FUNCTION "Uscite" : VOID
TITLE =Uscite
//Gestisce ed abilita le uscite
VERSION : 0.1

BEGIN
NETWORK
TITLE =Ultilità
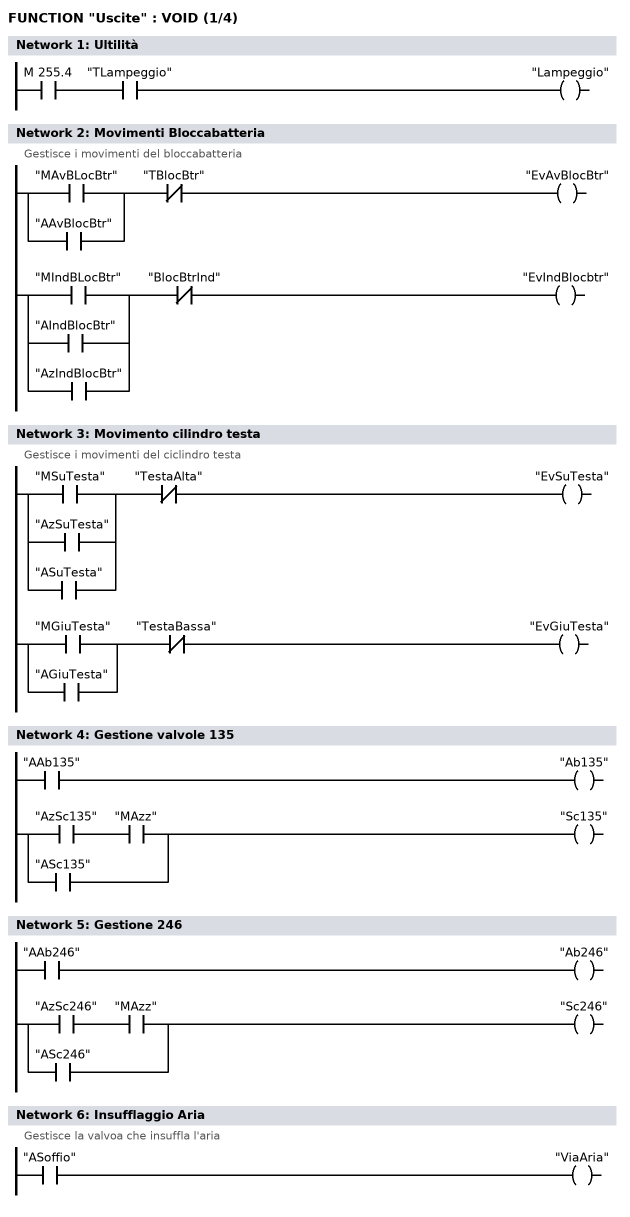
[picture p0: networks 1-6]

      U     M    255.4;
      U     "TLampeggio";
      =     "Lampeggio";



NETWORK
TITLE =Movimenti Bloccabatteria
//Gestisce i movimenti del bloccabatteria
      O     "MAvBLocBtr";
      O     "AAvBlocBtr";
      UN    "TBlocBtr";
      =     "EvAvBlocBtr";

      O     "MIndBLocBtr";
      O     "AIndBlocBtr";
      O     "AzIndBlocBtr";
      UN    "BlocBtrInd";
      =     "EvIndBlocbtr";


NETWORK
TITLE =Movimento cilindro testa
//Gestisce i movimenti del ciclindro testa
//
      O     "MSuTesta";
      O     "AzSuTesta";
      O     "ASuTesta";
      UN    "TestaAlta";
      =     "EvSuTesta";


      O     "MGiuTesta";
      O     "AGiuTesta";
      UN    "TestaBassa";
      =     "EvGiuTesta";


NETWORK
TITLE =Gestione valvole 135

//      ON    "MAzz"
      O     "AAb135";
      =     "Ab135";

      O(    ;
      U     "AzSc135";
      U     "MAzz";
      )     ;
      O     "ASc135";
      =     "Sc135";


NETWORK
TITLE =Gestione 246

//     On     "MAzz"
      O     "AAb246";
      =     "Ab246";



      O(    ;
      U     "AzSc246";
      U     "MAzz";
      )     ;
      O     "ASc246";
      =     "Sc246";



NETWORK
TITLE =Insufflaggio Aria
//Gestisce la valvoa che insuffla l'aria
      U     "ASoffio";
      =     "ViaAria";


NETWORK
TITLE =Lettura Batteria
//Valvola lettura batteria
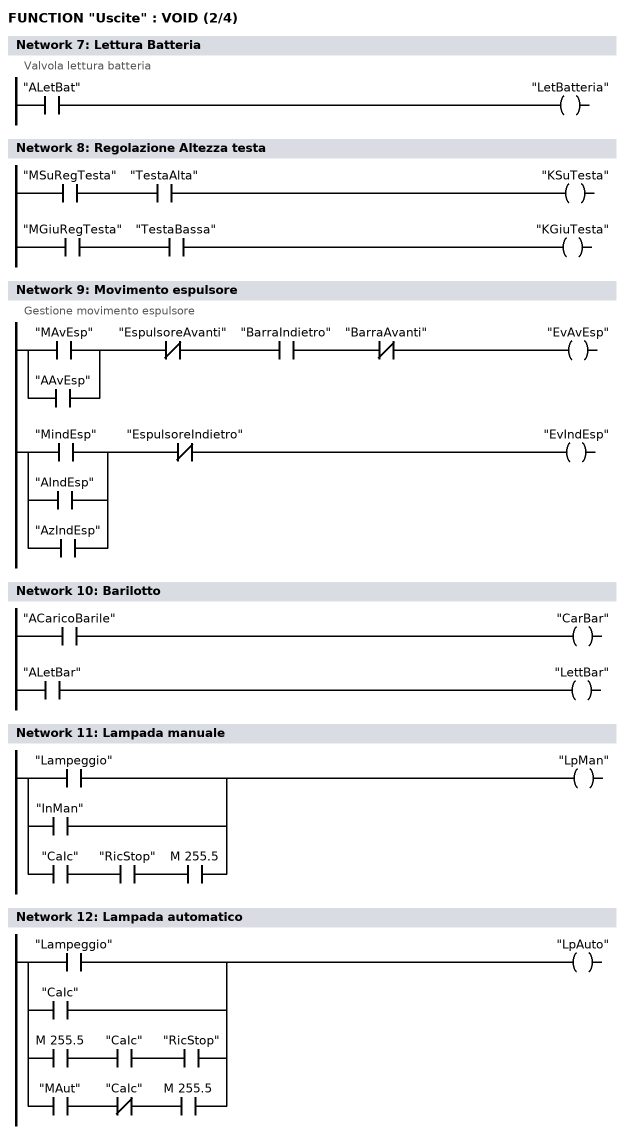
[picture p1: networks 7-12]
      U     "ALetBat";
      =     "LetBatteria";


NETWORK
TITLE =Regolazione Altezza testa

      U     "MSuRegTesta";
      U     "TestaAlta";
      =     "KSuTesta";

      U     "MGiuRegTesta";
      U     "TestaBassa";
      =     "KGiuTesta";


NETWORK
TITLE =Movimento espulsore
//Gestione movimento espulsore
      U(    ;
      O     "MAvEsp";
      O     "AAvEsp";
      )     ;
      UN    "EspulsoreAvanti";
      U     "BarraIndietro";
      UN    "BarraAvanti";
      =     "EvAvEsp";

      U(    ;
      O     "MindEsp";
      O     "AIndEsp";
      O     "AzIndEsp";
      )     ;
      UN    "EspulsoreIndietro";
      =     "EvIndEsp";


NETWORK
TITLE =Barilotto


      U     "ACaricoBarile";
      =     "CarBar";

      U     "ALetBar";
      =     "LettBar";


NETWORK
TITLE =Lampada manuale

      O     "Lampeggio";
      O     "InMan";
      O(    ;
      U     "CaIc";
      U     "RicStop";
      U     M    255.5;
      )     ;
      =     "LpMan";


NETWORK
TITLE =Lampada automatico

      O     "Lampeggio";
      O     "CaIc";
      O(    ;
      U     M    255.5;
      U     "CaIc";
      U     "RicStop";
      )     ;
      O(    ;
      U     "MAut";
      UN    "CaIc";
      U     M    255.5;
      )     ;
      =     "LpAuto";


NETWORK
TITLE =lampada macchina pronta
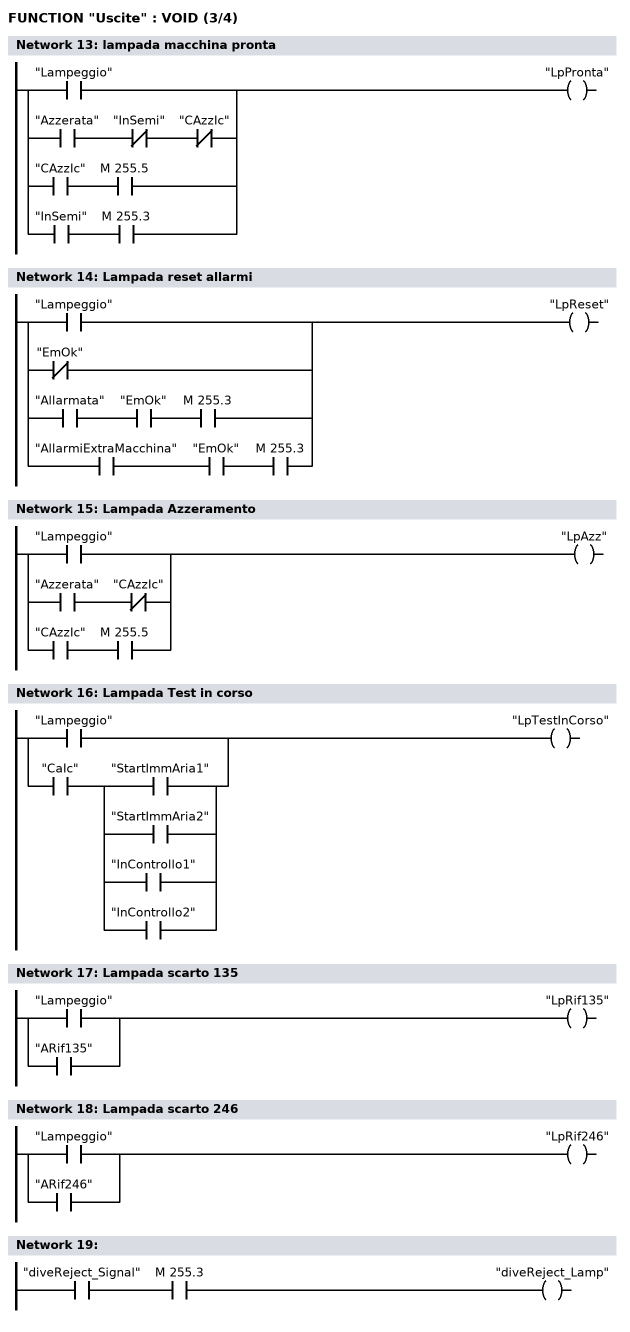
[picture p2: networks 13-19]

      O     "Lampeggio";
      O(    ;
      U     "Azzerata";
      UN    "InSemi";
      UN    "CAzzIc";
      )     ;
      O(    ;
      U     "CAzzIc";
      U     M    255.5;
      )     ;
      O(    ;
      U     "InSemi";
      U     M    255.3;
      )     ;
      =     "LpPronta";


NETWORK
TITLE =Lampada reset allarmi

      O     "Lampeggio";
      ON    "EmOk";
      O(    ;
      U     "Allarmata";
      U     "EmOk";
      U     M    255.3;
      )     ;
      O(    ;
      U     "AllarmiExtraMacchina";
      U     "EmOk";
      U     M    255.3;
      )     ;

      =     "LpReset";


NETWORK
TITLE =Lampada Azzeramento

      O     "Lampeggio";
      O(    ;
      U     "Azzerata";
      UN    "CAzzIc";
      )     ;
      O(    ;
      U     "CAzzIc";
      U     M    255.5;
      )     ;
      =     "LpAzz";
NETWORK
TITLE =Lampada Test in corso

      O     "Lampeggio";
      O(    ;
      U     "CaIc";
      U(    ;
      O     "StartImmAria1";
      O     "StartImmAria2";
      O     "InControllo1";
      O     "InControllo2";
      )     ;
      )     ;
      =     "LpTestInCorso";


NETWORK
TITLE =Lampada scarto 135

      O     "Lampeggio";
      O     "ARif135";
      =     "LpRif135";


NETWORK
TITLE =Lampada scarto 246

      O     "Lampeggio";
      O     "ARif246";
      =     "LpRif246";


NETWORK
TITLE =

      U     "diveReject_Signal";
      U     M    255.3;
      =     "diveReject_Lamp";

NETWORK
TITLE =Avviatore Progressivo
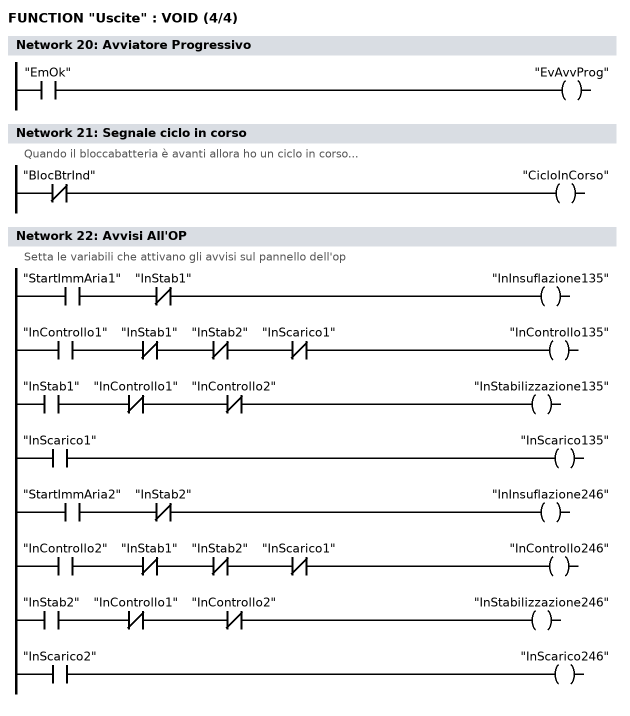
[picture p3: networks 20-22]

      U     "EmOk";
      =     "EvAvvProg";


NETWORK
TITLE =Segnale ciclo in corso
//Quando il bloccabatteria è avanti allora ho un ciclo in corso...
      UN    "BlocBtrInd";
      =     "CicloInCorso";

NETWORK
TITLE =Avvisi All'OP
//Setta le variabili che attivano gli avvisi sul pannello dell'op
      U     "StartImmAria1";
      UN    "InStab1";
      =     "InInsuflazione135";

      U     "InControllo1";
      UN    "InStab1";
      UN    "InStab2";
      UN    "InScarico1";
      =     "InControllo135";

      U     "InStab1";
      UN    "InControllo1";
      UN    "InControllo2";
      =     "InStabilizzazione135";

      U     "InScarico1";
      =     "InScarico135";

      U     "StartImmAria2";
      UN    "InStab2";
      =     "InInsuflazione246";

      U     "InControllo2";
      UN    "InStab1";
      UN    "InStab2";
      UN    "InScarico1";
      =     "InControllo246";


      U     "InStab2";
      UN    "InControllo1";
      UN    "InControllo2";
      =     "InStabilizzazione246";

      U     "InScarico2";
      =     "InScarico246";

END_FUNCTION

